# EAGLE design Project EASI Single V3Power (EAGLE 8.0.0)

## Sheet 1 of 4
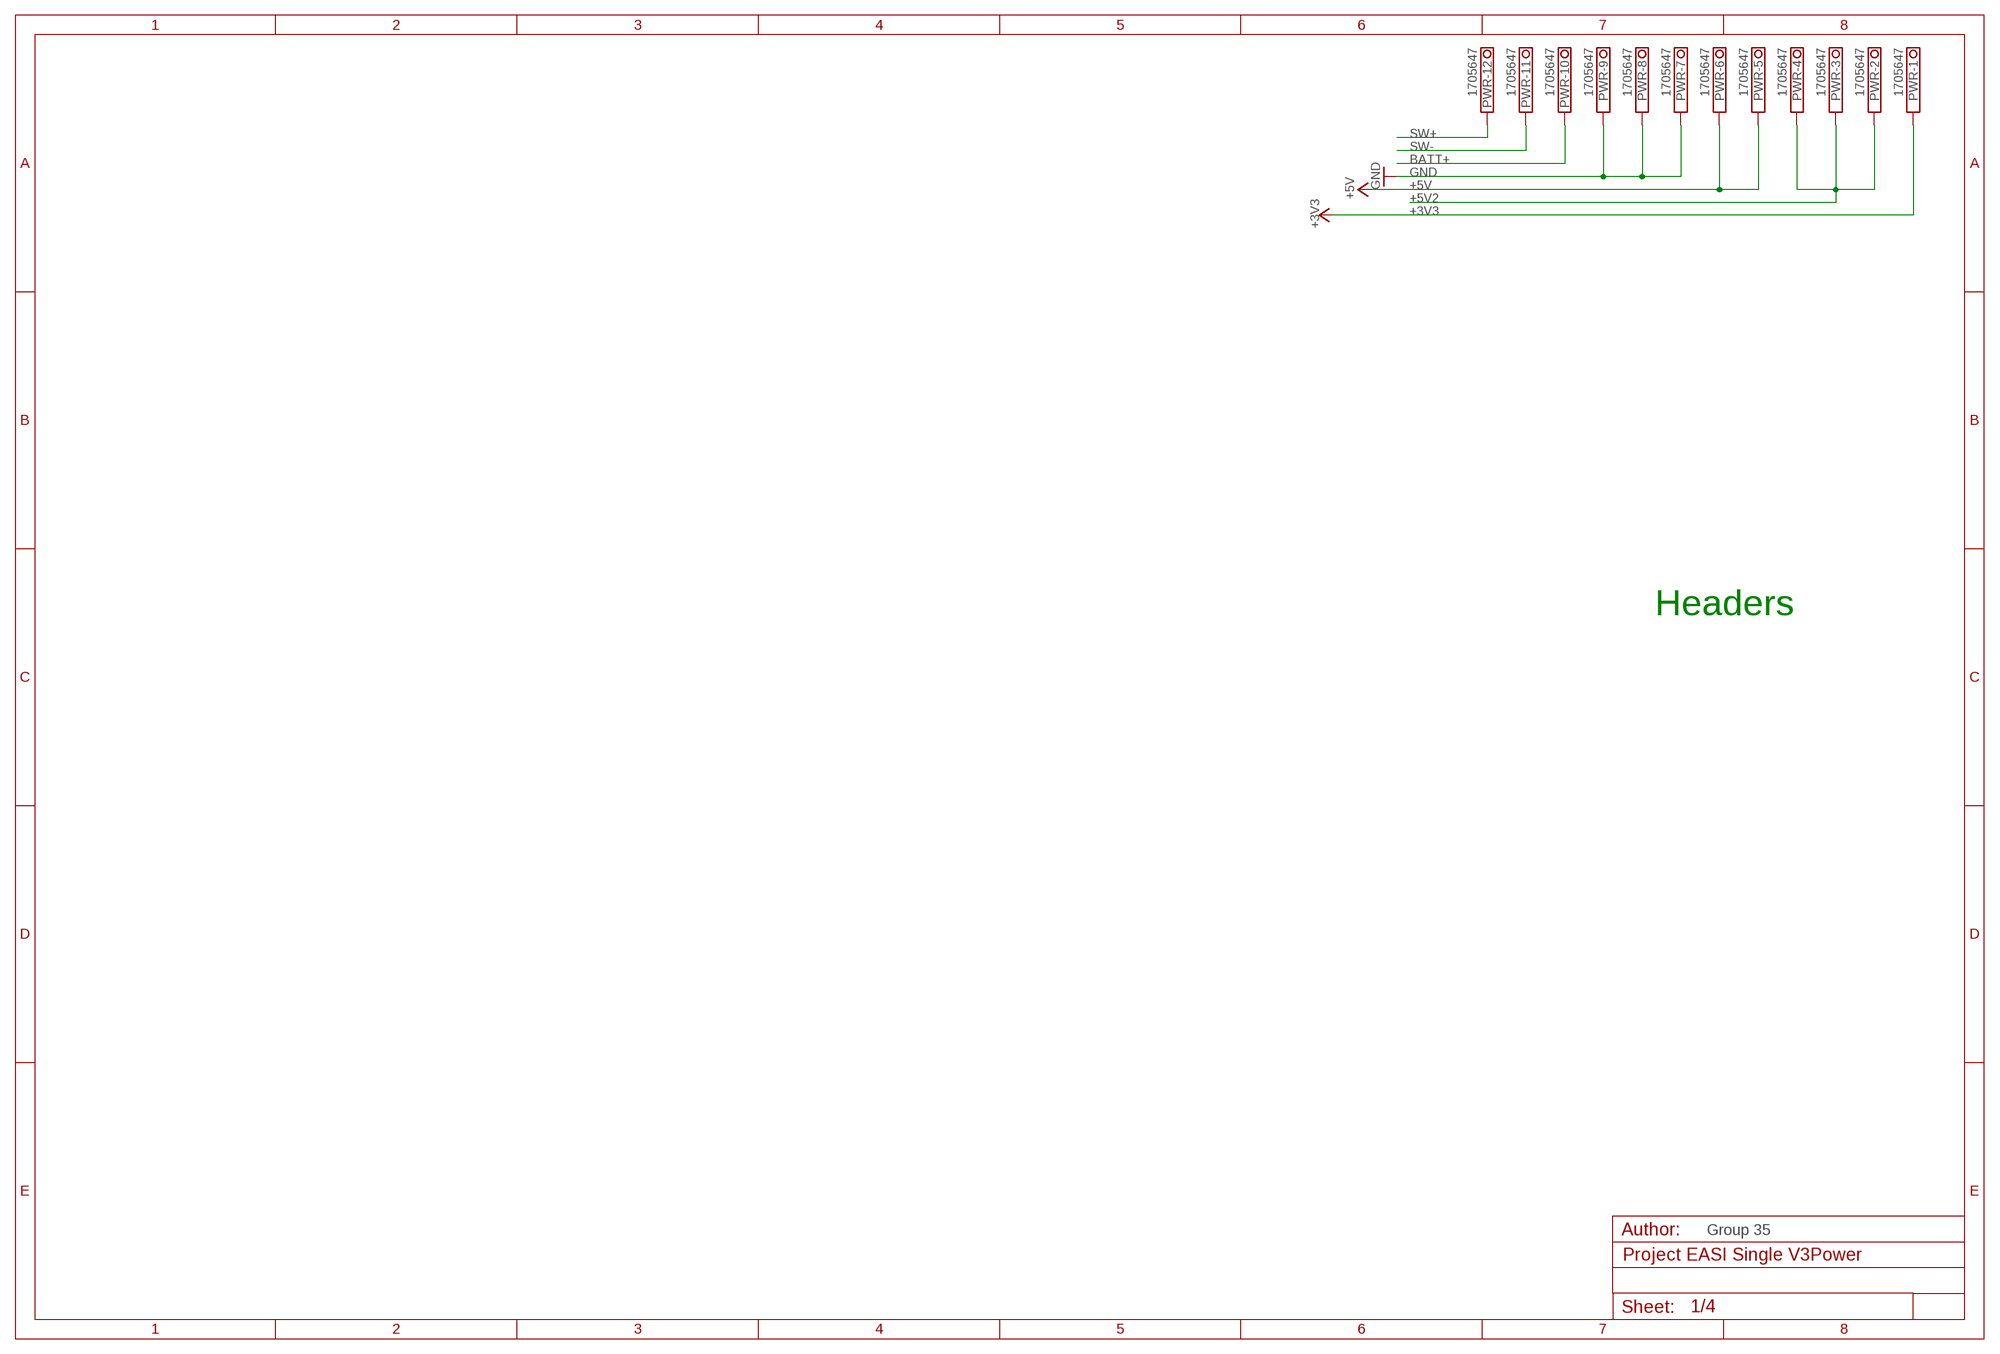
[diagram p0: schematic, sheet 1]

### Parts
PWR  1705647  [1705647]

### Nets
+3V3: PWR.1.1 PWR.1.2 ; also sheet 3
+5V: PWR.5.1 PWR.5.2 PWR.6.1 PWR.6.2 ; also sheet 3
+5V2: PWR.2.1 PWR.2.2 PWR.3.1 PWR.3.2 PWR.4.1 PWR.4.2 ; also sheet 3
BATT+: PWR.10.1 PWR.10.2 ; also sheet 3
GND [gnd]: PWR.7.1 PWR.7.2 PWR.8.1 PWR.8.2 PWR.9.1 PWR.9.2 ; also sheet 3
SW+: PWR.12.1 PWR.12.2 ; also sheet 3
SW-: PWR.11.1 PWR.11.2 ; also sheet 3

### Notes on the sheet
- Headers
- Group 35

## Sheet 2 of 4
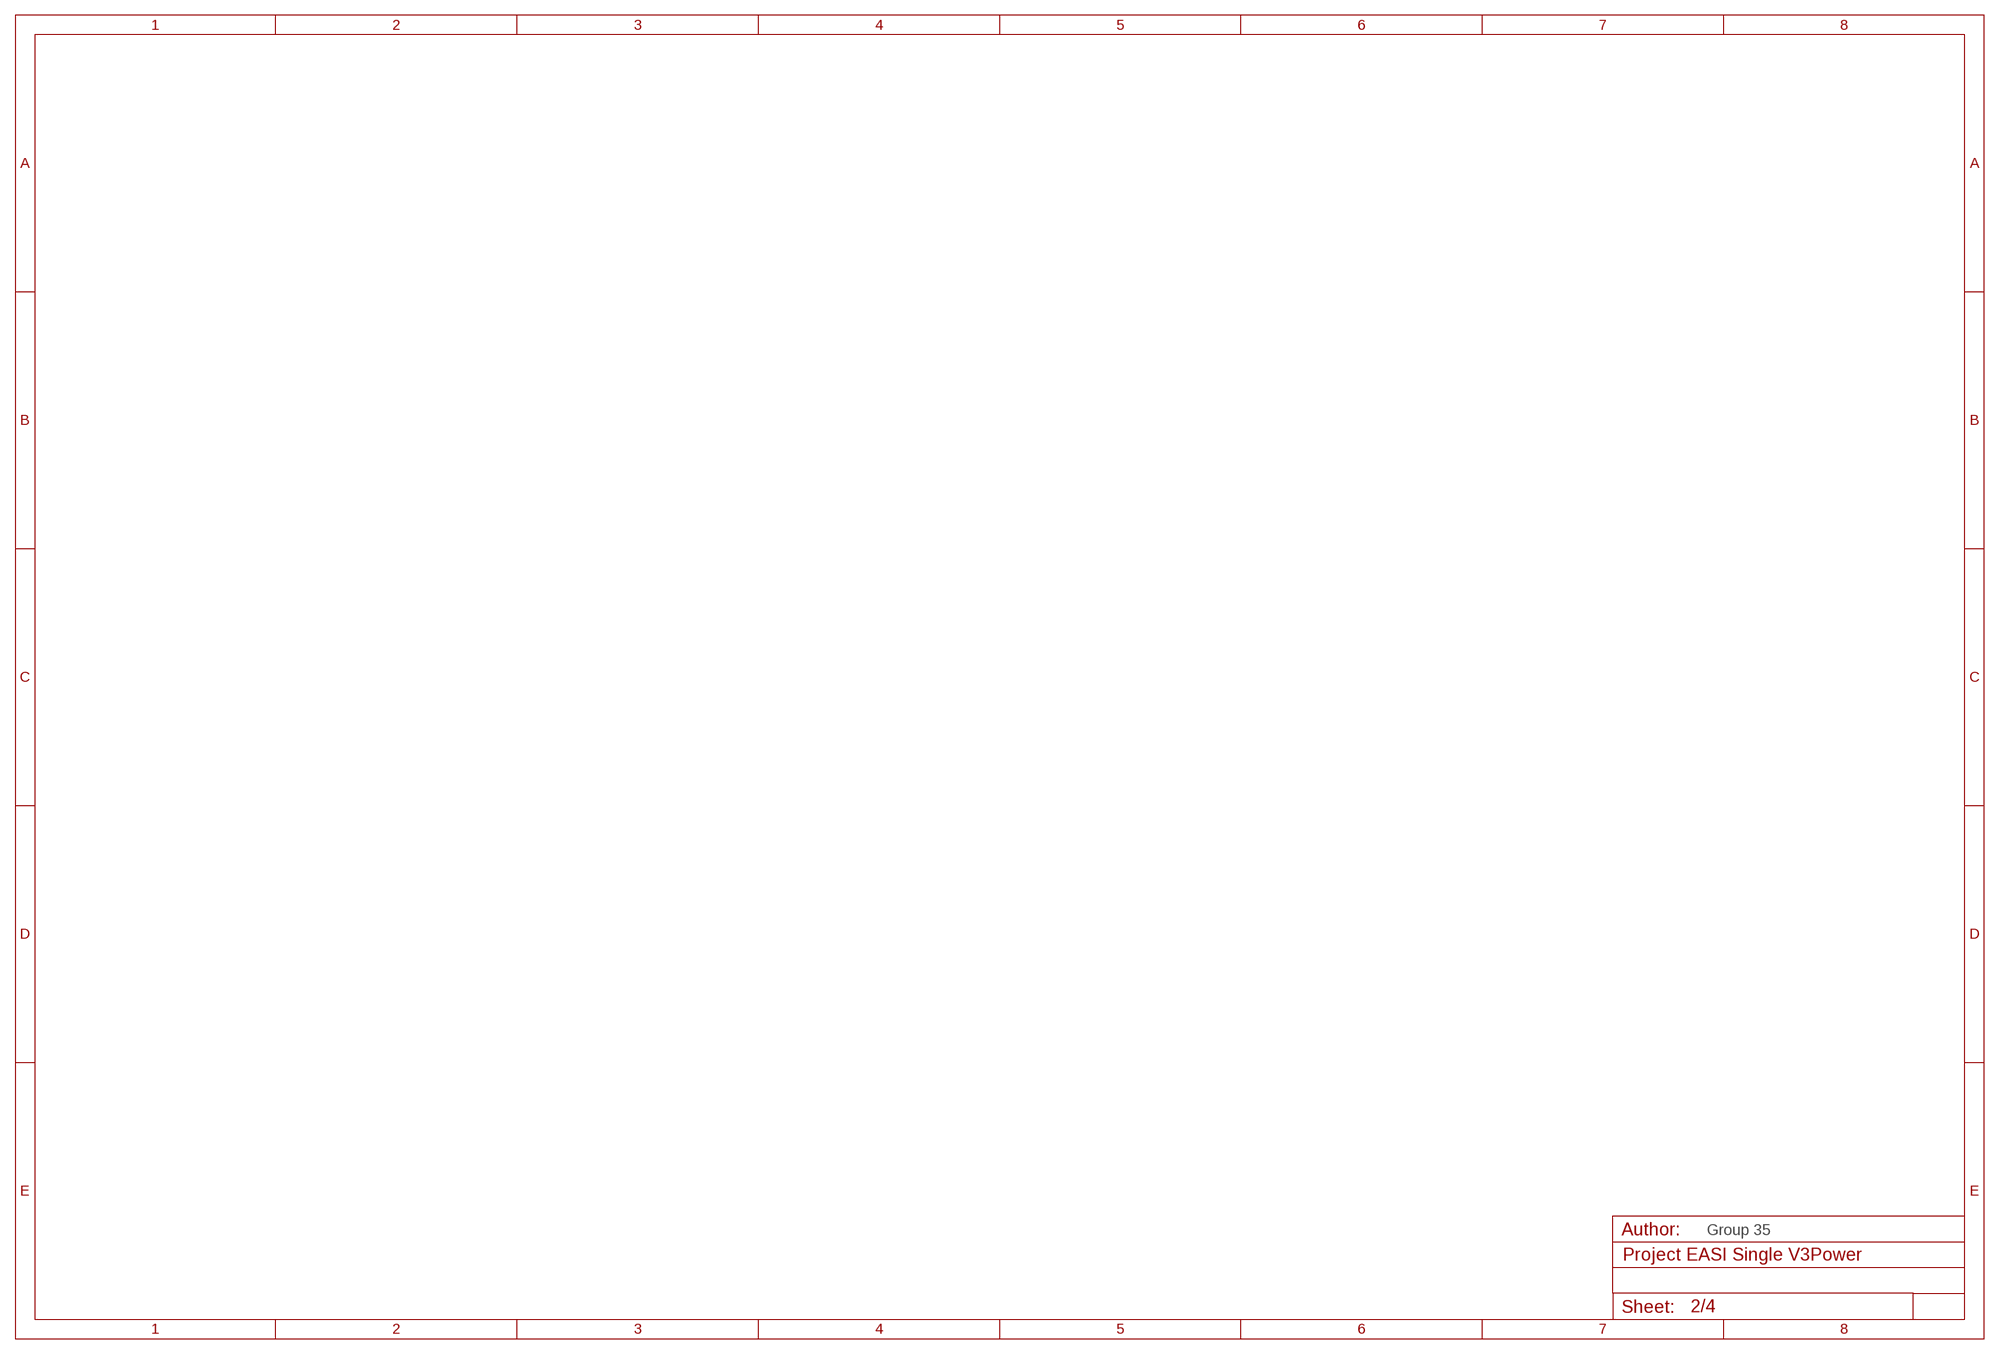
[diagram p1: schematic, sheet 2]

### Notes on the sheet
- Group 35

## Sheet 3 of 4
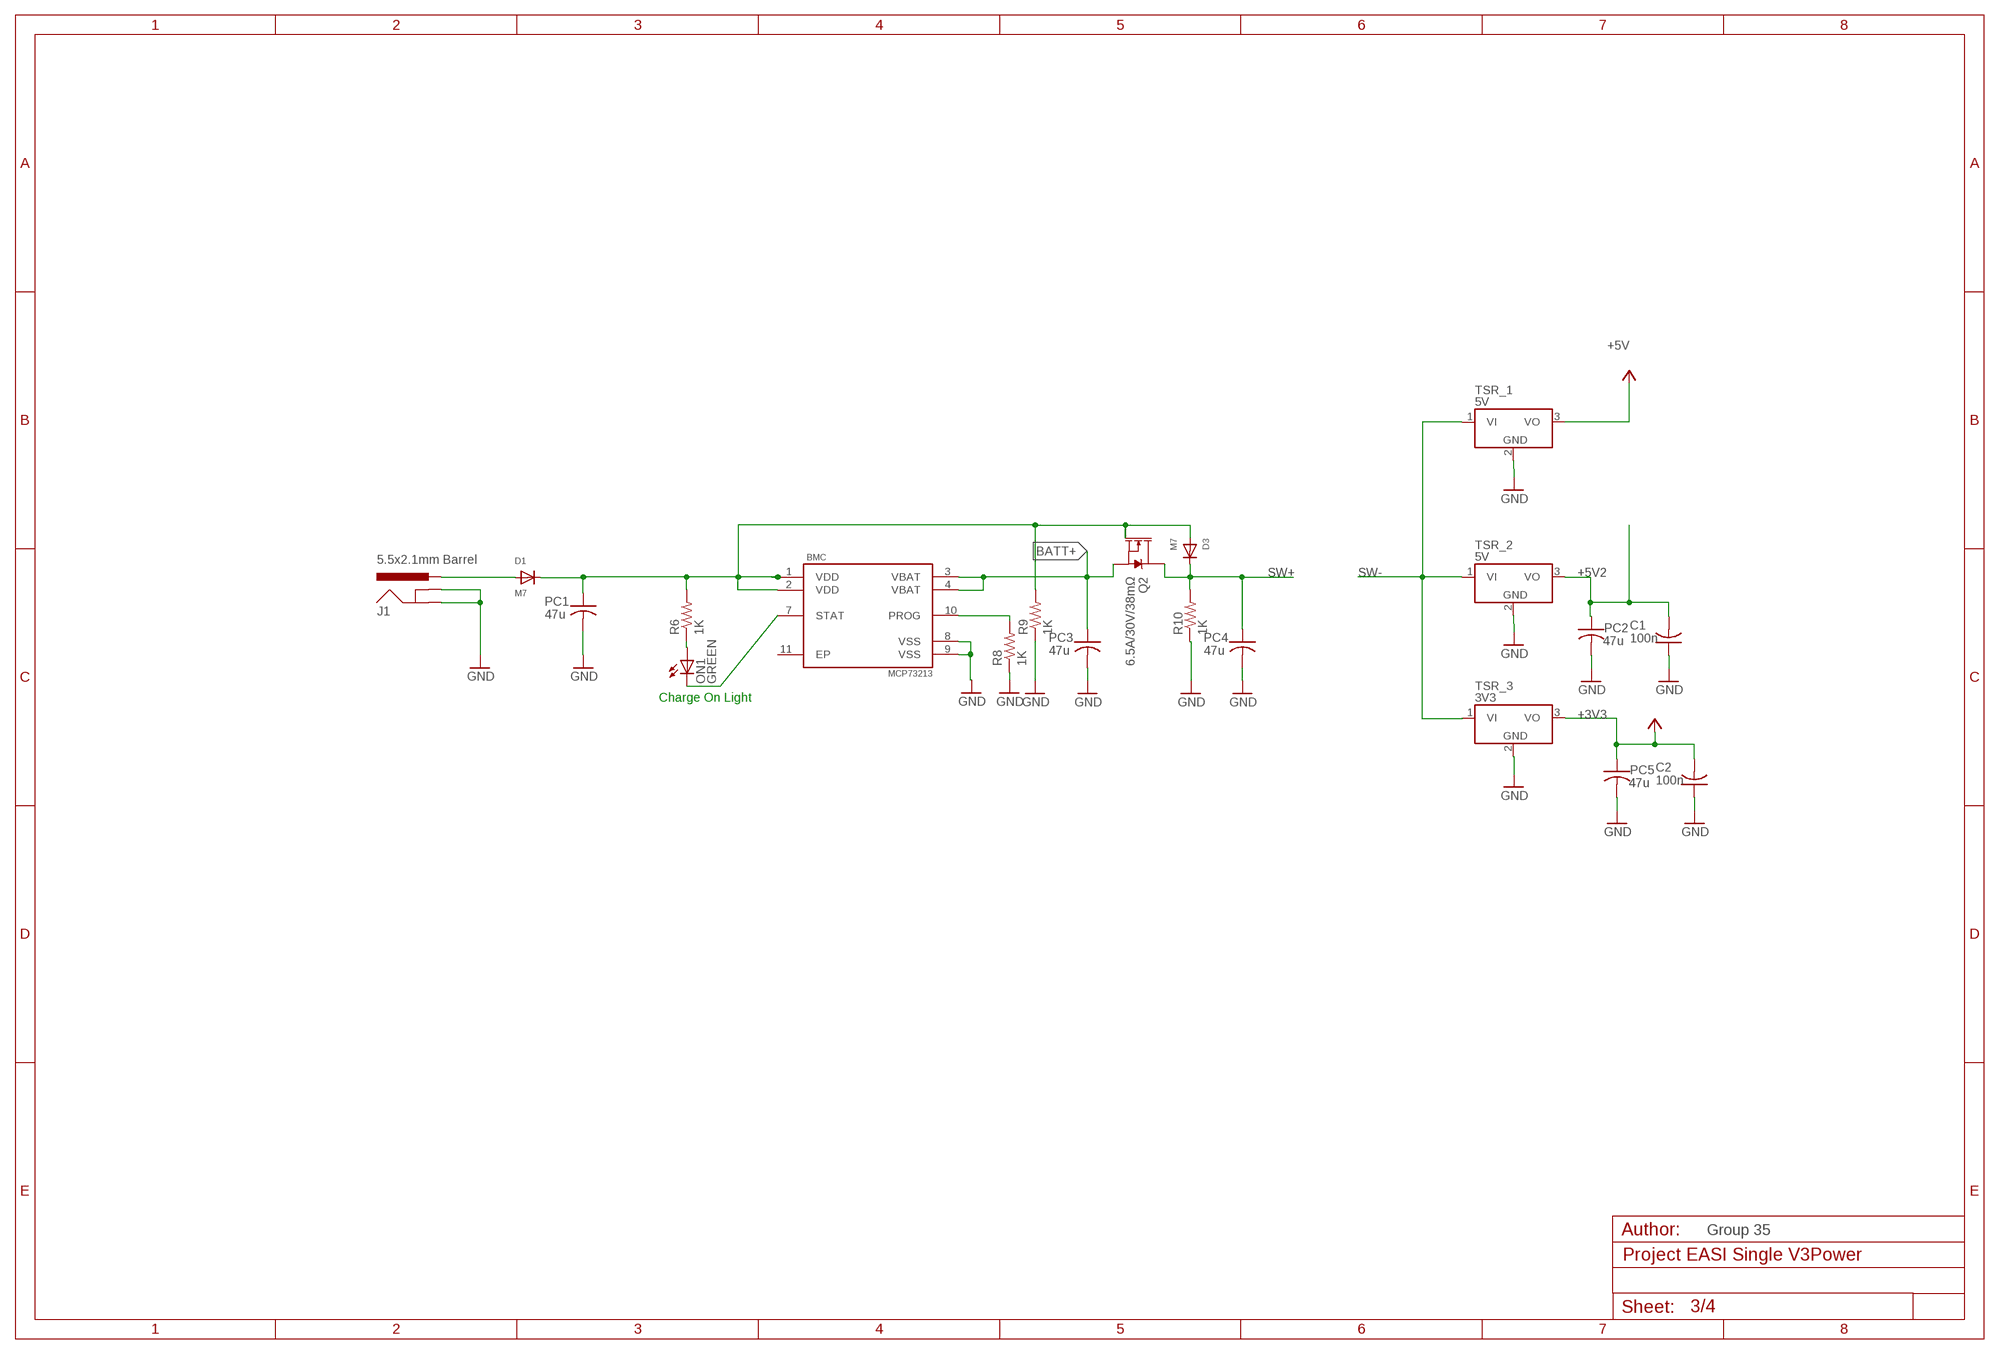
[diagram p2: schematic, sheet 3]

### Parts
BMC  MCP73213  [MCP73213]
C1  100n  C-USC0805  [C0805]
C2  100n  C-USC0805  [C0805]
D1  M7  DIODESMA  [SMADIODE]
D3  M7  DIODESMA  [SMADIODE]
J1  5.5x2.1mm Barrel  POWER_JACKSMD  [POWER_JACK_SMD]
ON1  GREEN  LEDCHIP-LED0805  [CHIP-LED0805]
PC1  47u  C-USC1206  [C1206]
PC2  47u  C-USC1206  [C1206]
PC3  47u  C-USC1206  [C1206]
PC4  47u  C-USC1206  [C1206]
PC5  47u  C-USC1206  [C1206]
Q2  6.5A/30V/38mΩ  MOSFET-NCH-FDS6630A  [SO08]
R6  1K  R-US_R0805  [R0805]
R8  1K  R-US_R0805  [R0805]
R9  1K  R-US_R0805  [R0805]
R10  1K  R-US_R0805  [R0805]
TSR_1  5V  TSR_1-24_  [TSR-1]
TSR_2  5V  TSR_1-24_  [TSR-1]
TSR_3  3V3  TSR_1-24_  [TSR-1]

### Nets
+3V3: C2.2 PC5.1 TSR_3.3(VO) ; also sheet 1
+5V: TSR_1.3(VO) ; also sheet 1
+5V2: C1.2 PC2.1 TSR_2.3(VO) ; also sheet 1
BATT+: BMC.3(VBAT) BMC.4(VBAT) PC3.1 Q2.1(S) Q2.2(S) Q2.3(S) ; also sheet 1
GND [gnd]: BMC.8(VSS) BMC.9(VSS) C1.1 C2.1 J1.GND(GNDBREAK) J1.P$4(GND) PC1.2 PC2.2 PC3.2 PC4.2 PC5.2 R8.1 R9.1 R10.1 TSR_1.2(GND) TSR_2.2(GND) TSR_3.2(GND) ; also sheet 1
N$2: D1.A J1.VIN0(PWR)
N$6: ON1.A R6.1
N$11: BMC.10(PROG) R8.2
N$13: BMC.7(STAT) ON1.C
N$29: BMC.1(VDD) BMC.2(VDD) D1.C D3.A PC1.1 Q2.4(G) R6.2 R9.2
SW+: D3.C PC4.1 Q2.5(D) Q2.6(D) Q2.7(D) Q2.8(D) R10.2 ; also sheet 1
SW-: TSR_1.1(VI) TSR_2.1(VI) TSR_3.1(VI) ; also sheet 1
Unconnected: BMC.11(EP)

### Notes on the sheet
- Charge On Light
- Group 35

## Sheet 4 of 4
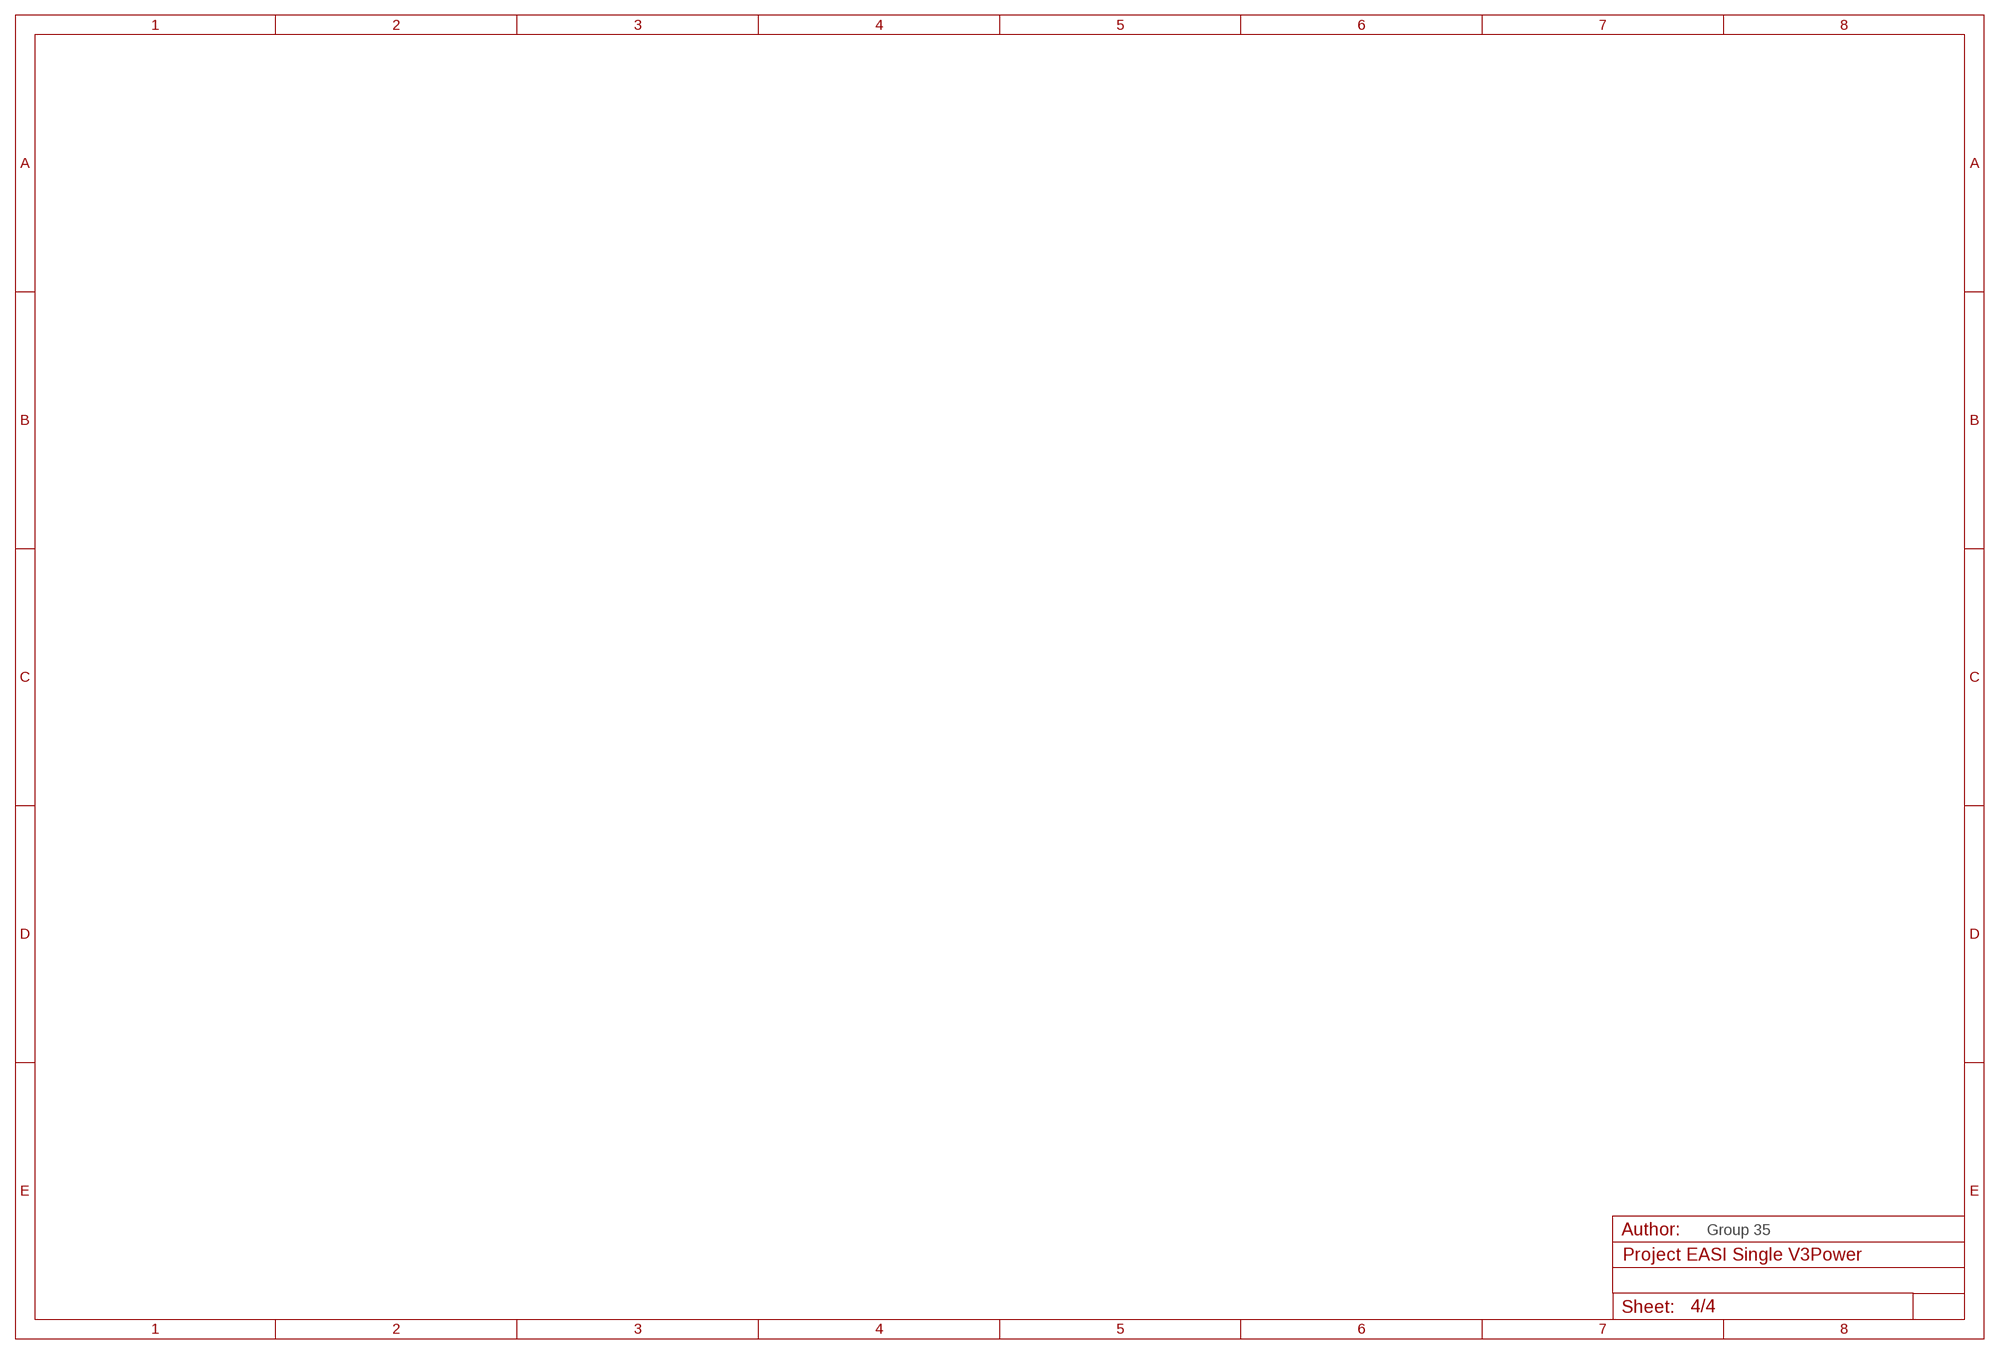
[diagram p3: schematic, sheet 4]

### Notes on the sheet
- Group 35

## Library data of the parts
BMC = Project_EASI_P_DualM_V1:MCP73213; MPN: MCP73213EV-2SOVP; OC_NEWARK: 26R1748
C1 C2 PC1-PC5 = adafruit:C-US: CAPACITOR, American symbol; OC_NEWARK: unknown
D1 D3 = microbuilder:DIODE: Diode; OC_NEWARK: unknown
J1 = SparkFun-Connectors:POWER_JACK: Power Jack Connector This is the standard 5.5mm barrel jack for power. The PTH is the most common, proven, reliable, footprint. The Slot footprint only works if the mill layer is transmitted to the PCB fab house so be warned. Here are the connectors we sell at SparkFun: DC Barrel Power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; OC_NEWARK: unknown; PROD_ID: CONN-08106; SF_ID: PRT-12748
ON1 = led:LED: LED; OC_NEWARK: unknown
PWR = con-phoenix-3.81-bigdrill holes:1705647: MKDSD 1,5/12-3,81 Printklemme Nennstrom: 8 A Bemessungsspannung: 200 V Raster: 3,81 mm Polzahl: 12 Montageart: Löten Anschlussart: Schraubanschluss Anschlussrichtung vom Leiter zur Platine: 0° Source: http://eshop.phoenixcontact.com .. 1705647.pdf; OC_FARNELL: unknown; OC_NEWARK: unknown
Q2 = SparkFun-DiscreteSemi:MOSFET-NCH: N-channel MOSFETs Voltage controlled devices that allow control of high current outputs. SparkFun Products: SparkFun OpenScale SparkFun Digital Sandbox SparkFun Monster Moto Shield SparkFun MOSFET Power Controller; OC_NEWARK: unknown; PROD_ID: TRANS-08089
R6 R8-R10 = adafruit:R-US_: RESISTOR, American symbol; OC_NEWARK: unknown
TSR_1-TSR_3 = _traco_tsr-1:TSR_1-*: TRACO TSR-1 Series Point-of-Load DC/DC-Converters Vi max. 36 V; Vo = (1.2 .. 15)V &plusmn;2%; Io = 0 .. 1 A SIP-Package (drop-in replacement for 78xx linear voltage regulators in TO220-package, vertically assembled) Source: www.tracopower.com Technologies: TSR 1- Vi (V) Vo (V) &plusmn;2% Io = 0 ..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; OC_NEWARK: unknown

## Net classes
0 default: width 0.203 mm, drill 5 mm, clearance 0.203 mm
1 USB: width 0.203 mm, drill 5 mm, clearance 0.203 mm to class 0
2 gnd: width 0.203 mm, drill 5 mm, clearance 0.203 mm to class 0
3 usbvcc: width 0.203 mm, drill 5 mm, clearance 0.203 mm to class 0, clearance 0.15 mm
4 USBpair: width 0.203 mm, drill 5 mm, clearance 0.203 mm to class 0, clearance 0.15 mm to class 3

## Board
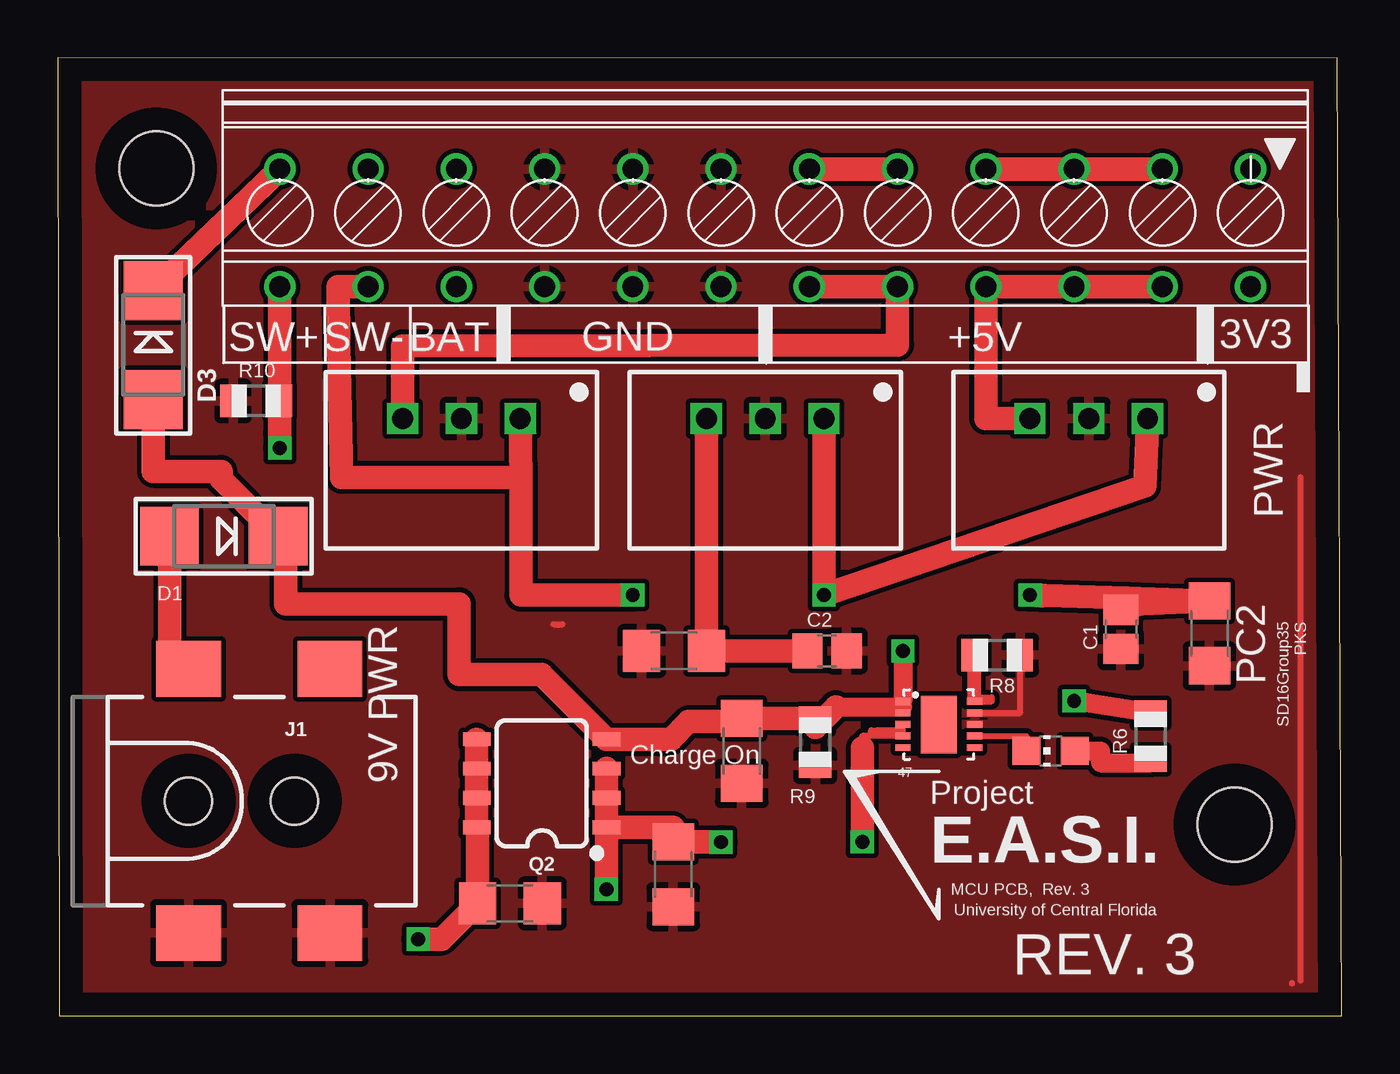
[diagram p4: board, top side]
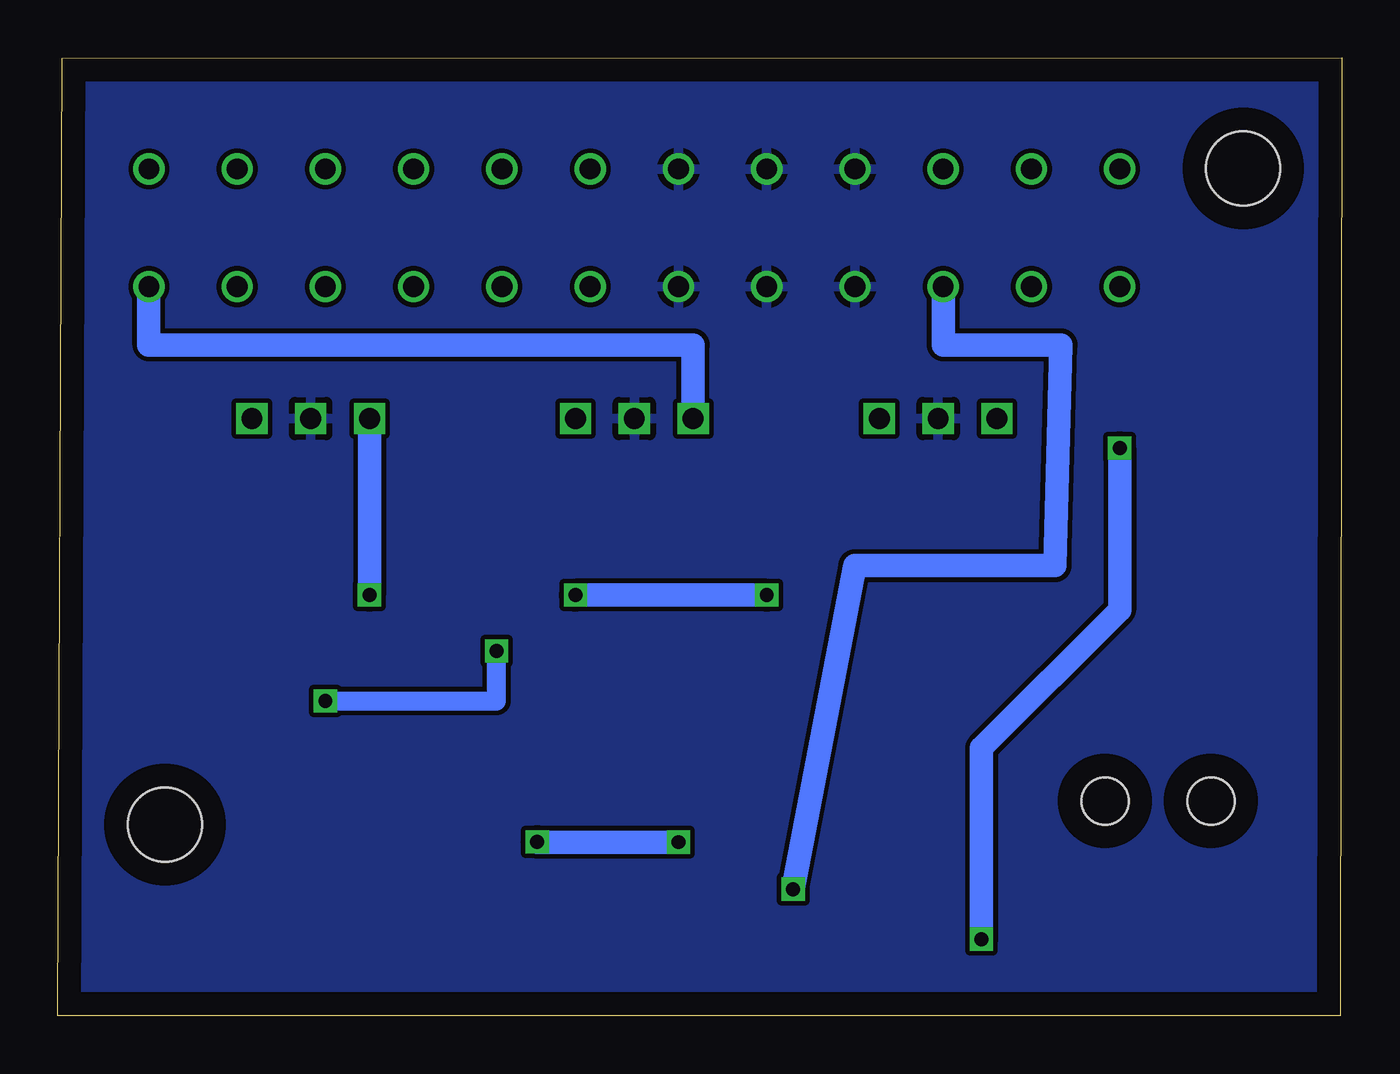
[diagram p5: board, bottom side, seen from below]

Size 55.42 x 41.35 mm. Coordinates in mm from the lower left corner, seen from the top.
Outline: 0.05,0 55.42,0.01 55.23,41.34 0,41.35 0.05,0
Copper layers (1*16): Top 0.035mm / dielectric 1.5mm / Bottom 0.035mm
Design rules "default *": minimum track width 10mil, minimum drill 15mil, track to track 8mil, track to pad 8mil, pad to pad 8mil, via to via 8mil, smd to smd 8mil, copper to edge 40mil, drill to drill 8mil, minimum pad ring 8mil, minimum via ring 8mil, stop-mask expansion 4mil, vias tented up to drill 0mil, thermal gap 10mil
Holes 3.2 mm at 50.79,8.25 4.24,36.58

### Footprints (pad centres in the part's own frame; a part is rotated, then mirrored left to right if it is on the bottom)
MCP73213 = smd 0.65 x 0.3: 1 -1.55,1; 2 -1.55,0.5; 3 -1.55,0; 4 -1.55,-0.5; 5 -1.55,-1; 6 1.55,-1; 7 1.55,-0.5; 8 1.55,0; 9 1.55,0.5; 10 1.55,1 | smd 1.55 x 2.48: 11 0,0
C0805 = smd 1.3 x 1.5: 1 -0.85,0; 2 0.85,0
SMADIODE = smd 2.54 x 2.54: A 2.349,0; C -2.349,0
POWER_JACK_SMD = smd 2.8 x 2.4: GND 0,-5.7; P$4 6.1,-5.7; VIN0 0,5.7; VIN1 6.1,5.7 | hole 2.032: 0,0; 4.572,0
CHIP-LED0805 = smd 1.2 x 1.2: A 0,-1.05; C 0,1.05
C1206 = smd 1.6 x 1.8: 1 -1.4,0; 2 1.4,0
1705647 = drill 0.9: 1.1 -20.955,-1.25; 1.2 -20.955,3.83; 2.1 -17.145,-1.25; 2.2 -17.145,3.83; 3.1 -13.335,-1.25; 3.2 -13.335,3.83; 4.1 -9.525,-1.25; 4.2 -9.525,3.83; 5.1 -5.715,-1.25; 5.2 -5.715,3.83; 6.1 -1.905,-1.25; 6.2 -1.905,3.83; 7.1 1.905,-1.25; 7.2 1.905,3.83; 8.1 5.715,-1.25; 8.2 5.715,3.83; 9.1 9.525,-1.25; 9.2 9.525,3.83; 10.1 13.335,-1.25; 10.2 13.335,3.83; 11.1 17.145,-1.25; 11.2 17.145,3.83; 12.1 20.955,-1.25; 12.2 20.955,3.83
SO08 = smd 0.6 x 1.2: 1 -1.905,-2.8; 2 -0.635,-2.8; 3 0.635,-2.8; 4 1.905,-2.8; 5 1.905,2.8; 6 0.635,2.8; 7 -0.635,2.8; 8 -1.905,2.8
R0805 = smd 1.1 x 1.4: 1 -1,0; 2 1,0
TSR-1 = drill 0.9 square: 1 -2.54,0; 2 0,0; 3 2.54,0

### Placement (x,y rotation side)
BMC  38.03,12.57 0 top
C1  45.89,16.68 90 top
C2  33.2,15.75 180 top
D1  7.17,20.7 180 top
D3  4.12,28.96 270 top
J1  5.64,9.27 0 top
ON1  42.85,11.43 90 top
PC1  29.52,11.43 270 top
PC2  49.71,16.51 270 top
PC3  26.56,6.11 270 top
PC4  19.51,4.85 0 top
PC5  26.6,15.75 180 top
PWR  30.53,35.31 180 top
Q2  20.88,10.03 90 top
R6  47.17,12.06 90 top
R8  40.55,15.57 180 top
R9  32.69,11.81 90 top
R10  8.56,26.54 0 top
TSR_1  17.42,25.78 180 top
TSR_2  44.5,25.78 180 top
TSR_3  30.53,25.78 180 top

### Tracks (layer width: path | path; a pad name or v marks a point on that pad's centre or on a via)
+3V3
  Top 1.016: TSR_3.3 PC5.1 C2.2
  Bottom 1.016: TSR_3.3 27.99,28.96 51.49,28.96 PWR.1.2
+5V
  Top 1.016: PWR.6.1 PWR.5.1 | TSR_1.3 14.88,28.91 36.25,28.96 PWR.5.2 PWR.6.2
+5V2  (via drill 0.6)
  Top 1.016: 42.47,18.12 v41.96,18.16 46.15,18.03 PC2.1 46.78,17.78 C1.2 | PWR.4.1 PWR.3.1 PWR.2.1 47.68,36.58 | PWR.2.2 PWR.3.2 PWR.4.2 40.06,25.78 TSR_2.3
  Bottom 1.016: TSR_2.3 v41.96,18.16
BATT+  (via drill 0.6)
  Top 0.254: 34.72,11.56 34.72,12.07 BMC.4 BMC.3 36.38,12.32 35.36,12.32 | 35.36,12.32 35.11,12.32 35.11,12.19 35.36,12.19 35.36,12.32
  Top 1.016: v23.68,5.46 Q2.1 | Q2.1 Q2.2 Q2.3 | Q2.1 26.55,8.13 PC3.1 28.63,7.51 v28.63,7.49 | v34.72,7.51 34.72,11.56
  Bottom 1.016: v23.68,5.46 21.01,19.43 12.37,19.43 12.12,28.96 17.2,28.96 PWR.10.2 | v28.63,7.49 34.72,7.49 v34.72,7.51
GND
  Top 0.254: 21.39,16.89 21.77,16.89 | 53.27,1.4 | 53.65,1.52 53.65,23.24 | BMC.9 41.55,13.07 R8.1
  pour Bottom: -5.03,83.82 148.64,83.82 148.64,-3.81 -5.03,-3.81
  pour Top: -8.84,86.36 168.96,86.36 168.96,-8.89 -8.84,-8.89
N$2
  Top 1.016: D1.A 4.82,15.8 J1.VIN0
N$6
  Top 0.813: ON1.A 45.01,11.43 45.01,10.92 47.17,10.92 R6.1
N$11
  Top 0.254: BMC.10 40.31,13.57 40.31,13.75 39.55,13.75
  Top 0.61: R8.2 39.55,13.75
N$13
  Top 0.254: BMC.7 41.8,12.07 ON1.C
N$29  (via drill 0.6)
  Top 0.254: BMC.2 36.48,13.34 BMC.1
  Top 0.813: 33.58,13.34 36.48,13.34 | R6.2 v43.87,13.59 | v36.48,15.74 BMC.1
  Top 1.016: D3.A 4.12,23.5 7.04,23.5 7.04,23.18 D1.C 9.83,20.7 9.83,17.78 17.33,17.78 17.33,14.73 20.89,14.73 Q2.4 26.47,11.94 27.23,12.7 29.27,12.7 PC1.1 32.55,12.83 R9.2 32.69,12.45 33.58,13.34
  Bottom 0.813: v43.87,13.59 36.48,13.59 v36.48,15.74
SW+  (via drill 0.6)
  Top 1.016: PWR.12.2 9.56,31.48 R10.2 | R10.2 9.56,25.15 | PWR.12.1 arc-90 9.47,36.45 D3.C | R10.2 9.56,24.53 v9.58,24.51 | v15.55,3.3 16.56,3.3 PC4.1 18.11,8.1 Q2.8 Q2.7 Q2.6 Q2.5
  Bottom 1.016: v9.58,24.51 9.58,17.53 15.55,11.56 v15.55,3.3
SW-  (via drill 0.6)
  Top 1.016: TSR_1.1 19.99,23.24 | 19.99,23.24 12.25,23.24 12.12,28.96 12.09,31.48 PWR.11.2 | 19.99,23.24 19.99,18.16 v24.82,18.16 | TSR_3.1 v33.07,18.16 46.92,22.86 TSR_2.1
  Bottom 1.016: v24.82,18.16 v33.07,18.16

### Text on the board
tPlace: SW+ | SW- | BAT | GND | +5V | 3V3 | SD16Group35 / PKS | 9V PWR | 47 | Project | E.A.S.I. | MCU PCB, Rev. 3 | University of Central Florida | REV. 3
tSilk: Charge On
